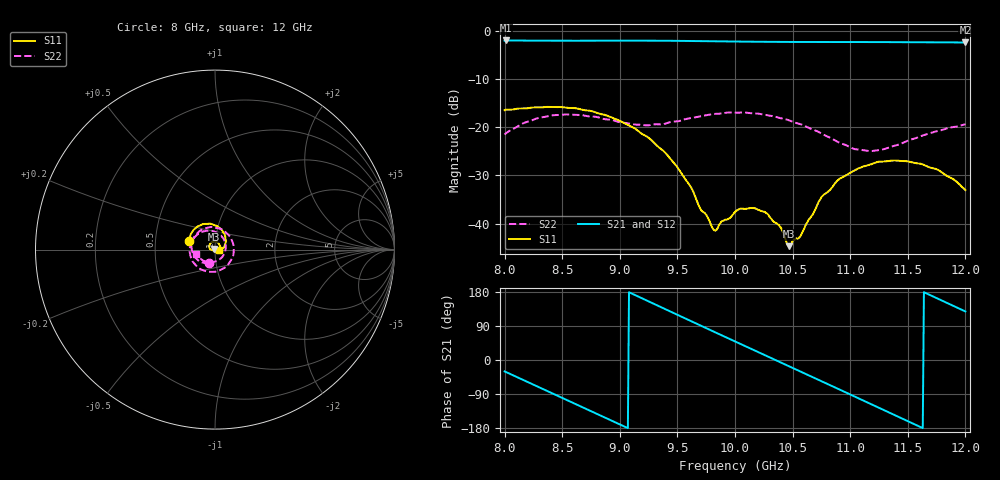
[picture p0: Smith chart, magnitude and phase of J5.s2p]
!Keysight Technologies,N5234A,MY52241180,A.10.60.03
!Date: Tuesday, May 30, 2023 15:22:55
!Correction: S11(Full 2 Port(1,2))
!S21(Full 2 Port(1,2))
!S12(Full 2 Port(1,2))
!S22(Full 2 Port(1,2))
!S2P File: Measurements: S11, S21, S12, S22:
# Hz S  dB  R 50
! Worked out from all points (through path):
!   401 points, 8 GHz to 12 GHz, reference 50 ohm
!   highest |S21| = -2.03 dB at 8.01 GHz (marker M1); lowest = -2.5 dB at 12 GHz (marker M2)
!   group delay of S21, straight-line fit = 390 ps
!   lowest |S11| = -44.7 dB at 10.47 GHz (marker M3), VSWR 1.01, Z = 49.6 + j0.371 ohm
!   |S11| at or under -10 dB: start of sweep to end of sweep
!   |S22| runs from -25.0 to -16.9 dB; largest |S21 - S12| = 0.0015
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8e9  -16.48 161.8  -2.09 -30.1  -2.09 -30.1  -21.54 -114.4
8.01e9  -16.39 161.5  -2.03 -31.4  -2.05 -31.5  -21.29 -116.4
8.35e9  -15.83 140.3  -2.09 -78.9  -2.09 -79.0  -17.86 -177.3
8.51e9  -15.87 125.9  -2.09 -101.2  -2.10 -101.2  -17.40 154.6
8.67e9  -16.37 109.9  -2.08 -123.6  -2.10 -123.6  -17.49 124.9
8.85e9  -17.34 90.0  -2.07 -148.8  -2.08 -148.9  -18.23 89.2
9.01e9  -18.78 70.3  -2.07 -171.3  -2.08 -171.4  -19.02 53.7
9.17e9  -20.99 50.0  -2.06 166.0  -2.08 166.0  -19.48 13.8
9.34e9  -24.18 26.3  -2.09 142.0  -2.09 141.9  -19.42 -29.9
9.58e9  -31.14 -15.8  -2.13 108.0  -2.14 108.0  -18.28 -85.9
9.82e9  -41.40 -116.5  -2.21 74.2  -2.21 74.2  -17.26 -133.0
1e10  -37.54 171.6  -2.26 49.0  -2.26 48.9  -17.01 -165.0
1.027e10  -37.81 131.0  -2.32 11.3  -2.32 11.2  -17.48 150.8
1.047e10  -44.65 140.2  -2.34 -16.6  -2.35 -16.7  -18.59 118.6
1.067e10  -38.25 -170.0  -2.35 -44.6  -2.36 -44.6  -20.45 83.8
1.076e10  -34.22 -174.2  -2.35 -57.2  -2.36 -57.3  -21.43 67.2
1.1e10  -29.45 161.6  -2.36 -90.9  -2.36 -91.0  -24.16 13.8
1.116e10  -27.87 137.7  -2.36 -113.5  -2.37 -113.5  -24.95 -28.1
1.134e10  -26.99 112.0  -2.37 -138.8  -2.38 -138.9  -24.17 -70.6
1.15e10  -27.09 86.4  -2.39 -161.4  -2.40 -161.4  -22.78 -102.6
1.166e10  -28.02 58.5  -2.41 176.0  -2.41 176.0  -21.48 -127.7
1.2e10  -33.03 -0.6  -2.45 128.1  -2.46 128.1  -19.39 -167.8
